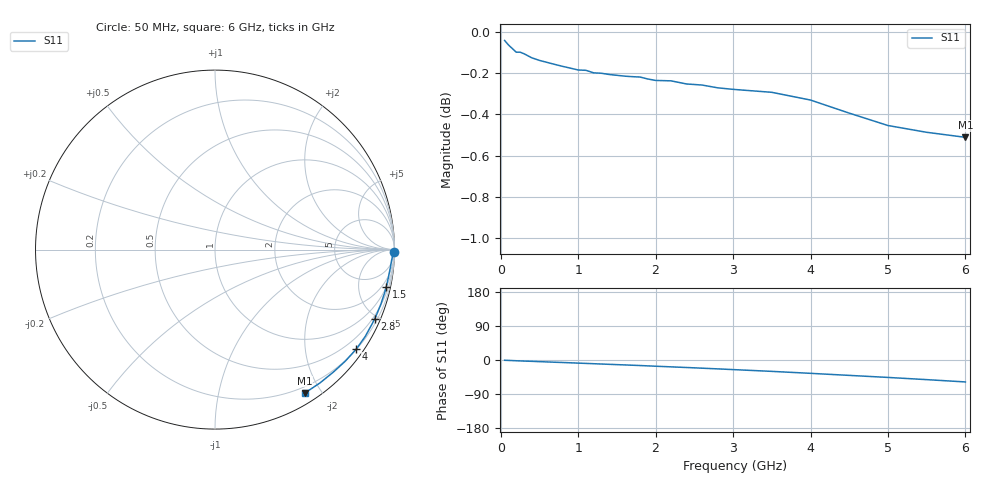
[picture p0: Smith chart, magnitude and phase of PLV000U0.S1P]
! Infineon Technologies  Discrete & RF Semiconductors
! BAR 64-04W /-05W /-06W
! Si PIN Diode in SOT323
! VR = 0 V
! S-Parameters:  October  2008
# GHz  S  MA  R  50
!  f  S11
! GHz  MAG  ANG
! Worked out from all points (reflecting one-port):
!   34 points, 50 MHz to 6 GHz, reference 50 ohm
!   lowest |S11| = -0.5 dB at 6 GHz (marker M1), VSWR 33.97, Z = 6.26 - j90.1 ohm
!   phase of S11 starts at -1 deg and turns -57 deg over the sweep
!   S11 on the Smith chart (normalised r, x): 50 MHz: open; 1.5 GHz: 1.06, -9.24; 2.8 GHz: 0.38, -4.80; 4 GHz: 0.21, -3.14; 6 GHz: 0.13, -1.80
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0.05  0.9953 -0.7
0.1  0.9928 -1.1
0.15  0.9908 -1.5
0.2  0.9888 -2.0
0.25  0.9888 -2.4
0.3  0.988 -2.8
0.4  0.9857 -3.5
0.7  0.982 -5.9
0.8  0.981 -6.6
1  0.979 -8.2
1.1  0.9788 -9.0
1.2  0.9775 -9.8
1.3  0.9772 -10.6
1.5  0.9761 -12.2
1.6  0.9756 -13.0
1.8  0.9752 -14.6
2  0.9733 -16.4
2.2  0.9731 -18.1
2.4  0.9714 -19.8
2.6  0.9708 -21.6
2.8  0.9693 -23.4
3  0.9685 -25.3
3.5  0.9669 -30.0
4  0.9627 -35.2
4.5  0.9557 -40.6
5  0.9491 -46.0
5.5  0.9455 -51.8
6  0.9428 -57.9
